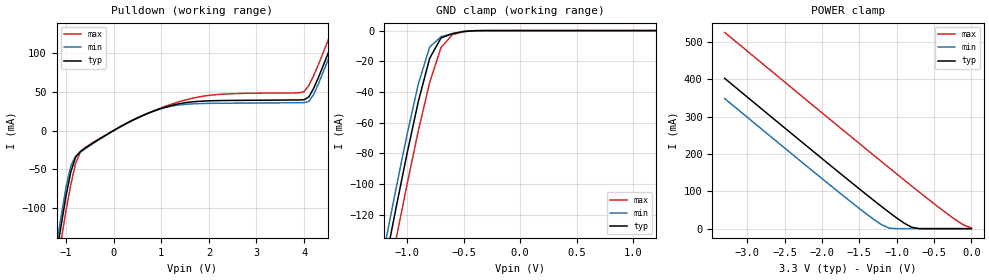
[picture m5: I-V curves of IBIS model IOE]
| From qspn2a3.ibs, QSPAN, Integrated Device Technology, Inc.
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|   Model IOE
[Model]   IOE
Model_type   I/O
Polarity   Non-Inverting
Vinl =   0.8000V
Vinh =   2.0000V
C_comp   5.0000pF   5.0000pF   5.0000pF
[Temperature Range]   27.0000   0.000   70.0000
[Voltage Range]   3.3000V   3.0000V   4.0000V
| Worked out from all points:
|   slope of the pulldown table from 0 to 0.495 V, typ, clamps not added: 30.8 ohm
|   GND clamp passes 1 mA (typ) near -0.53 V on its own axis
|   POWER clamp passes 1 mA (typ) near -0.72 V on its own axis
[Pulldown]
| voltage   I(typ)   I(min)   I(max)
-3.3V     -989.3mA   -977.6mA   -1.008A
-1.5V     -271mA     -258.5mA   -291.1mA
-1V       -83.95mA   -72.71mA   -103mA
-800mV    -34.25mA   -33.24mA   -42.4mA
-600mV    -22.73mA   -23.68mA   -21.99mA
800mV     24.09mA    24.25mA    24.39mA
2V        38.3mA     35.03mA    45.32mA
4V        39.69mA    36.03mA    50.22mA
4.2V      54.39mA    46.58mA    70.77mA
4.7V      130.8mA    122.8mA    147.4mA
4.9V      163.4mA    155.5mA    179.7mA
6.6V      454mA      447.8mA    466.7mA
[Pullup]
| voltage   I(typ)   I(min)   I(max)
-3.3V     0A         NA         NA
6.6V      0A         NA         NA
[GND_clamp]
| voltage   I(typ)   I(min)   I(max)
-3.3V     -989mA     -977.4mA   -1.007A
-1.2V     -154mA     -141.4mA   -174.5mA
-1.1V     -116.5mA   -103.8mA   -136.9mA
-1V       -80.1mA    -67.71mA   -100.2mA
-900mV    -46.07mA   -34.65mA   -65.22mA
-800mV    -18.04mA   -10.76mA   -33.77mA
-700mV    -4.837mA   -3.97mA    -11.11mA
-600mV    -2.032mA   -2.01mA    -2.705mA
-500mV    -595.8uA   -531.1uA   -729.2uA
-400mV    -67.77uA   -42.52uA   -120.1uA
1.2V      15.7pA     7.974pA    207pA
[POWER_clamp]
| voltage   I(typ)   I(min)   I(max)
-3.3V     402.4mA    348.3mA    525.5mA
-1.8V     155.3mA    101.9mA    277.5mA
-1.4V     90.64mA    38.72mA    211.8mA
-1.2V     59mA       10.41mA    179.2mA
-1.1V     43.57mA    1.444mA    162.9mA
-900mV    14.76mA    424.9nA    130.5mA
-800mV    3.845mA    6.104nA    114.4mA
-700mV    187.3uA    119pA      98.4mA
-200mV    43.97pA    28.09pA    22.07mA
-100mV    42.35pA    27.3pA     9.496mA
0V        41.54pA    26.52pA    1.592mA
[Ramp]
| variable   typ   min   max
dV/dt_r   0/0   0/0   0/0
dV/dt_f   1.0776/0.1236n   0.9864/0.1153n   1.2888/0.1264n
R_load = 50.0000
| End [Model] IOE
